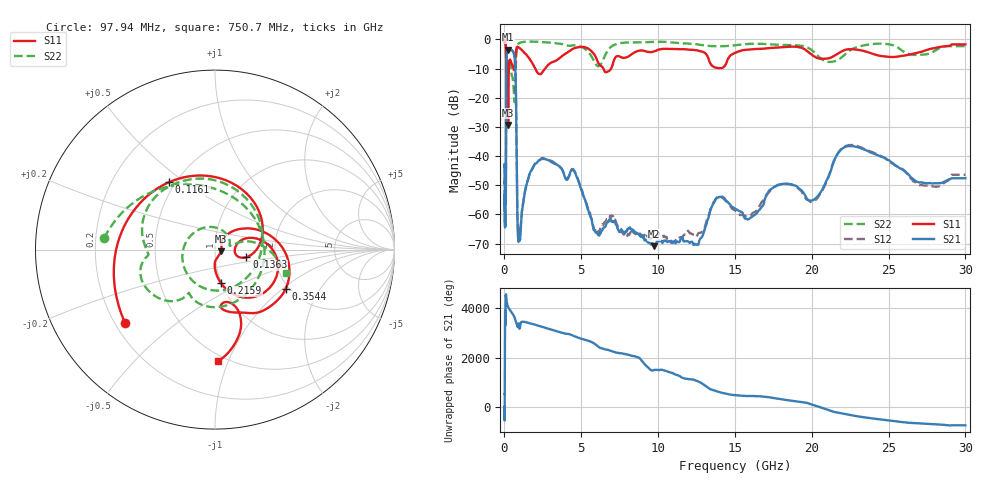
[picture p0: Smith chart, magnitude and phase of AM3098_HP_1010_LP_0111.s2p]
! Date/Time: Thu, Feb 28, 2019 8:42 AM
! Network Analyzer: Agilent Technologies E8364B Rev: A.07.50.67
! Sweep from 0.010 to 30.000 GHz, 1601 Points, Sweep Type: LOG
! Power Supply: 5.022 V, 0.002 A
# Hz S DB R 50
!freq MagS11 AngS11 MagS21 AngS21 MagS12 AngS12 MagS22 AngS22
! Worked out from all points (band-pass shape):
!   1601 points, 10 MHz to 30 GHz, reference 50 ohm
!   highest |S21| = -3.46 dB at 237.5 MHz (marker M1); lowest = -70.9 dB at 9.731 GHz (marker M2)
!   |S21| within 3 dB of the highest: 133 MHz to 665 MHz (532 MHz wide, 133 % of centre)
!   lowest |S11| = -29.3 dB at 238.7 MHz (marker M3), VSWR 1.07, Z = 53.4 - j1.06 ohm
!   |S11| at or under -10 dB: 200 MHz to 289.2 MHz (89.13 MHz wide, 36.4 % of centre); 2.01 GHz to 2.645 GHz (635.7 MHz wide, 27.3 % of centre); 6.44 GHz to 6.941 GHz (501.2 MHz wide, 7.49 % of centre)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
!   |S22| runs from -21.5 to -0.5 dB; largest |S21 - S12| = 0.014
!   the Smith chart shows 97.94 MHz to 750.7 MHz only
!   S11 on the Smith chart (normalised r, x): 97.94 MHz: 0.24, -0.34; 116.1 MHz: 0.46, +0.44; 136.3 MHz: 1.42, -0.12; 215.9 MHz: 1.00, -0.39; 354.4 MHz: 1.92, -1.05; 750.7 MHz: 0.45, -0.92
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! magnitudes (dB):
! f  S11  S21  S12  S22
! 10 MHz  -0.3  -43.6  -43.0  -0.5
! 38.04 MHz  -0.4  -59.6  -57.6  -0.9
! 97.94 MHz  -3.8  -47.6  -46.8  -4.1
! 116.1 MHz  -6.8  -18.7  -18.7  -10.9
! 136.3 MHz  -14.9  -5.8  -5.7  -10.7
! 144.7 MHz  -19.1  -4.8  -4.8  -10.9
! 215.9 MHz  -14.4  -3.6  -3.6  -8.1
! 237.5 MHz  -29.3  -3.5  -3.4  -8.6
! 238.7 MHz  -29.3  -3.5  -3.4  -8.6
! 354.4 MHz  -6.9  -3.8  -3.8  -7.4
! 550.5 MHz  -9.5  -4.1  -4.1  -13.9
! 750.7 MHz  -4.1  -19.6  -19.6  -7.6
! 842.3 MHz  -2.5  -60.8  -59.9  -2.2
! 912.5 MHz  -2.7  -68.4  -66.3  -1.4
! 2.084 GHz  -10.8  -42.4  -42.0  -0.8
! 4.503 GHz  -3.1  -44.9  -44.6  -2.0
! 5.959 GHz  -6.2  -66.2  -66.5  -8.6
! 7.926 GHz  -6.2  -65.9  -66.6  -1.1
! 9.731 GHz  -4.1  -70.9  -68.0  -0.8
! 20.1 GHz  -5.6  -55.0  -55.6  -4.1
! 22.56 GHz  -3.3  -36.6  -36.2  -3.5
! 30 GHz  -1.7  -47.6  -46.4  -2.3
